(* Logix 5000 AddOnInstructionDefinition export Banner_DFG1_Param_v4; software revision 32.00; part 2 of 2 *)
(* tags used below, declared in another part *)
   DFG1 : Banner_DFG1_v2;
   Port_Data : Banner_IOL_Port_v4;
   Port : DINT;
   Local_Control : DINT;
   Command_Being_Processed : BOOL;
   Update_Archive : BOOL;
   Index_Write_Inprocess : DINT;
   Inprocess_Index : DINT;
(* Banner_DFG1_Param_v4, continued *)

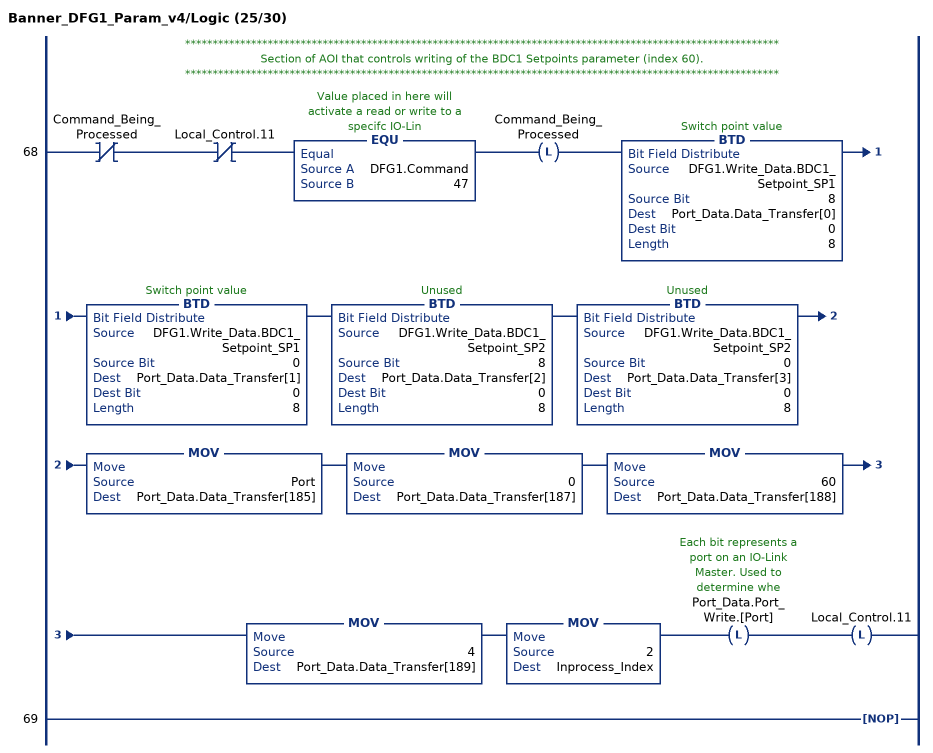
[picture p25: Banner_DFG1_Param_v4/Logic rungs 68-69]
   // ************************************************************************************************************
   // Section of AOI that controls writing of the BDC1 Setpoints parameter (index 60).
   // ************************************************************************************************************
   68: XIO(Command_Being_Processed)XIO(Local_Control.11)EQU(DFG1.Command,47)OTL(Command_Being_Processed)BTD(DFG1.Write_Data.BDC1_Setpoint_SP1,8,Port_Data.Data_Transfer[0],0,8)BTD(DFG1.Write_Data.BDC1_Setpoint_SP1,0,Port_Data.Data_Transfer[1],0,8)BTD(DFG1.Write_Data.BDC1_Setpoint_SP2,8,Port_Data.Data_Transfer[2],0,8)BTD(DFG1.Write_Data.BDC1_Setpoint_SP2,0,Port_Data.Data_Transfer[3],0,8)MOV(Port,Port_Data.Data_Transfer[185])MOV(0,Port_Data.Data_Transfer[187])MOV(60,Port_Data.Data_Transfer[188])MOV(4,Port_Data.Data_Transfer[189])MOV(2,Inprocess_Index)OTL(Port_Data.Port_Write.[Port])OTL(Local_Control.11);
   69: NOP();
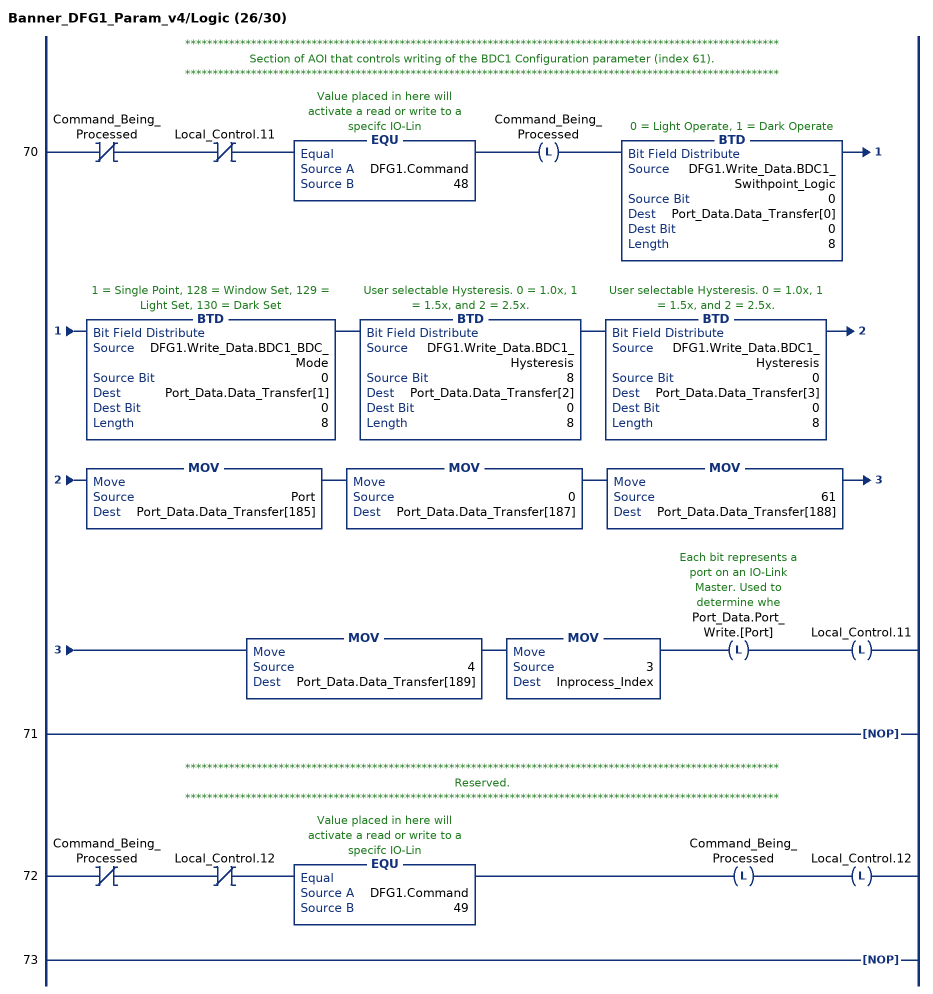
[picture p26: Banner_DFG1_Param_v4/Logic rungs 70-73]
   // ************************************************************************************************************
   // Section of AOI that controls writing of the BDC1 Configuration parameter (index 61).
   // ************************************************************************************************************
   70: XIO(Command_Being_Processed)XIO(Local_Control.11)EQU(DFG1.Command,48)OTL(Command_Being_Processed)BTD(DFG1.Write_Data.BDC1_Swithpoint_Logic,0,Port_Data.Data_Transfer[0],0,8)BTD(DFG1.Write_Data.BDC1_BDC_Mode,0,Port_Data.Data_Transfer[1],0,8)BTD(DFG1.Write_Data.BDC1_Hysteresis,8,Port_Data.Data_Transfer[2],0,8)BTD(DFG1.Write_Data.BDC1_Hysteresis,0,Port_Data.Data_Transfer[3],0,8)MOV(Port,Port_Data.Data_Transfer[185])MOV(0,Port_Data.Data_Transfer[187])MOV(61,Port_Data.Data_Transfer[188])MOV(4,Port_Data.Data_Transfer[189])MOV(3,Inprocess_Index)OTL(Port_Data.Port_Write.[Port])OTL(Local_Control.11);
   71: NOP();
   // ************************************************************************************************************
   // Reserved.
   // ************************************************************************************************************
   72: XIO(Command_Being_Processed)XIO(Local_Control.12)EQU(DFG1.Command,49)OTL(Command_Being_Processed)OTL(Local_Control.12);
   73: NOP();
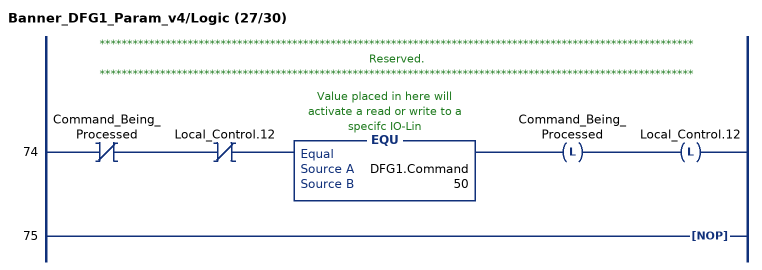
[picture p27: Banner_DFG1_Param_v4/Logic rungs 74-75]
   // ************************************************************************************************************
   // Reserved.
   // ************************************************************************************************************
   74: XIO(Command_Being_Processed)XIO(Local_Control.12)EQU(DFG1.Command,50)OTL(Command_Being_Processed)OTL(Local_Control.12);
   75: NOP();
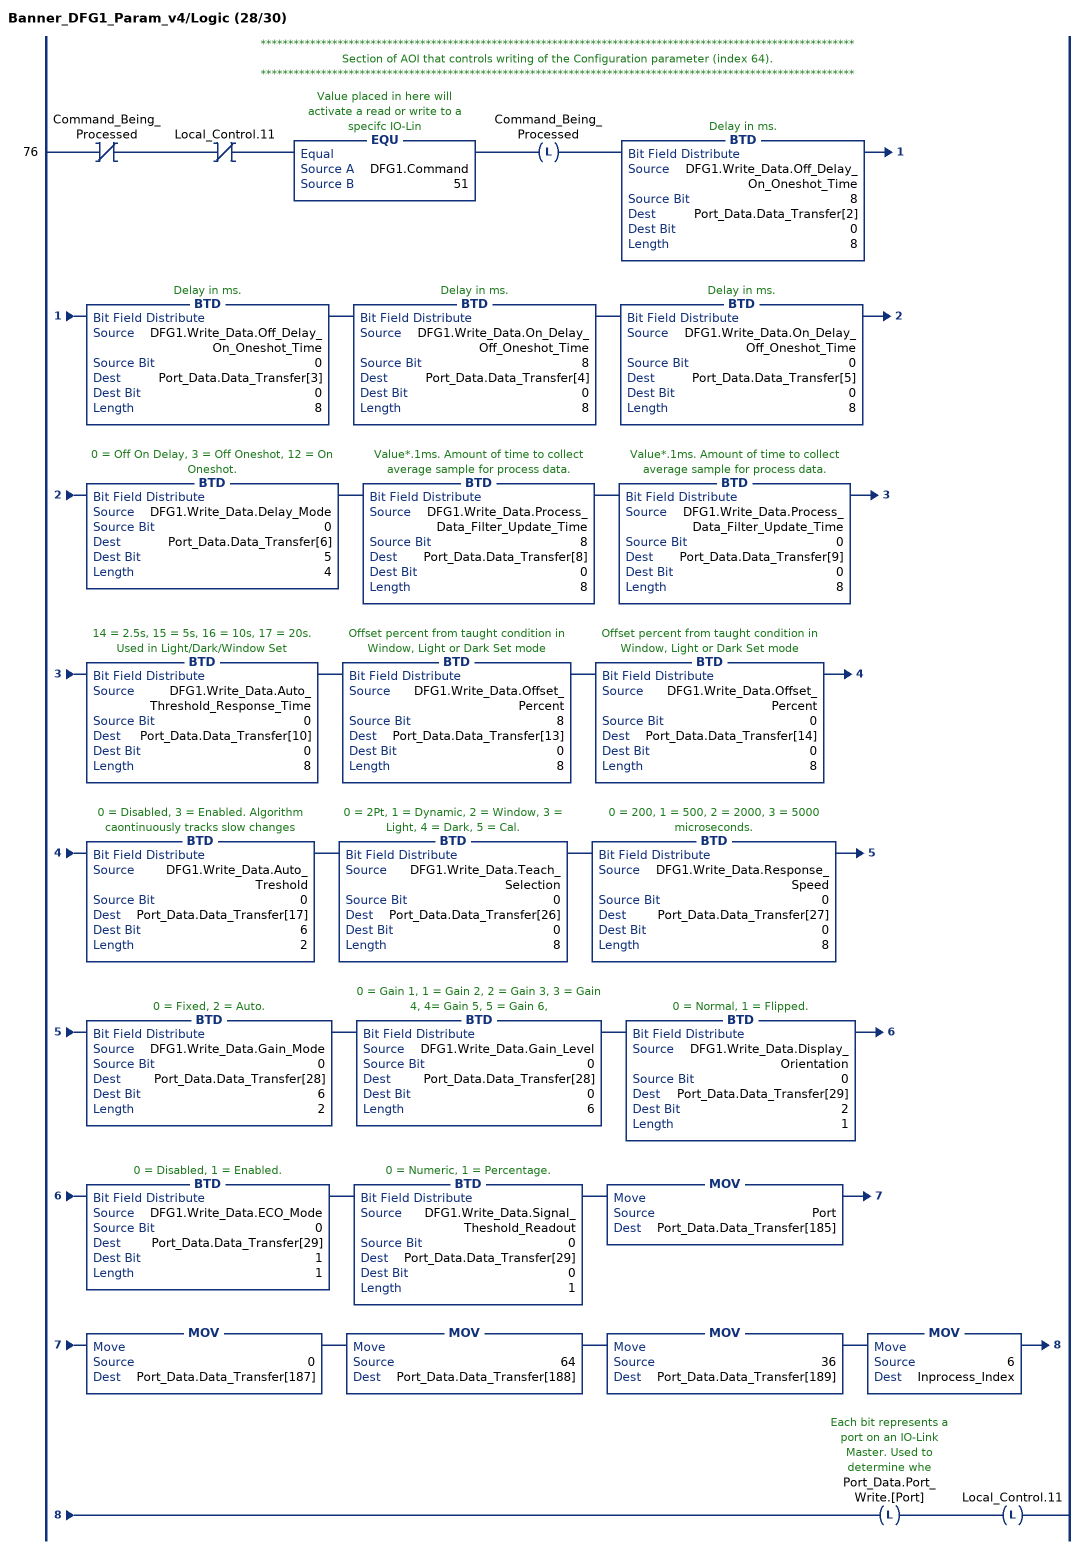
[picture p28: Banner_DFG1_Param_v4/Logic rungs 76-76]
   // ************************************************************************************************************
   // Section of AOI that controls writing of the Configuration parameter (index 64).
   // ************************************************************************************************************
   76: XIO(Command_Being_Processed)XIO(Local_Control.11)EQU(DFG1.Command,51)OTL(Command_Being_Processed)BTD(DFG1.Write_Data.Off_Delay_On_Oneshot_Time,8,Port_Data.Data_Transfer[2],0,8)BTD(DFG1.Write_Data.Off_Delay_On_Oneshot_Time,0,Port_Data.Data_Transfer[3],0,8)BTD(DFG1.Write_Data.On_Delay_Off_Oneshot_Time,8,Port_Data.Data_Transfer[4],0,8)BTD(DFG1.Write_Data.On_Delay_Off_Oneshot_Time,0,Port_Data.Data_Transfer[5],0,8)BTD(DFG1.Write_Data.Delay_Mode,0,Port_Data.Data_Transfer[6],5,4)BTD(DFG1.Write_Data.Process_Data_Filter_Update_Time,8,Port_Data.Data_Transfer[8],0,8)BTD(DFG1.Write_Data.Process_Data_Filter_Update_Time,0,Port_Data.Data_Transfer[9],0,8)BTD(DFG1.Write_Data.Auto_Threshold_Response_Time,0,Port_Data.Data_Transfer[10],0,8)BTD(DFG1.Write_Data.Offset_Percent,8,Port_Data.Data_Transfer[13],0,8)BTD(DFG1.Write_Data.Offset_Percent,0,Port_Data.Data_Transfer[14],0,8)BTD(DFG1.Write_Data.Auto_Treshold,0,Port_Data.Data_Transfer[17],6,2)BTD(DFG1.Write_Data.Teach_Selection,0,Port_Data.Data_Transfer[26],0,8)BTD(DFG1.Write_Data.Response_Speed,0,Port_Data.Data_Transfer[27],0,8)BTD(DFG1.Write_Data.Gain_Mode,0,Port_Data.Data_Transfer[28],6,2)BTD(DFG1.Write_Data.Gain_Level,0,Port_Data.Data_Transfer[28],0,6)BTD(DFG1.Write_Data.Display_Orientation,0,Port_Data.Data_Transfer[29],2,1)BTD(DFG1.Write_Data.ECO_Mode,0,Port_Data.Data_Transfer[29],1,1)BTD(DFG1.Write_Data.Signal_Theshold_Readout,0,Port_Data.Data_Transfer[29],0,1)MOV(Port,Port_Data.Data_Transfer[185])MOV(0,Port_Data.Data_Transfer[187])MOV(64,Port_Data.Data_Transfer[188])MOV(36,Port_Data.Data_Transfer[189])MOV(6,Inprocess_Index)OTL(Port_Data.Port_Write.[Port])OTL(Local_Control.11);
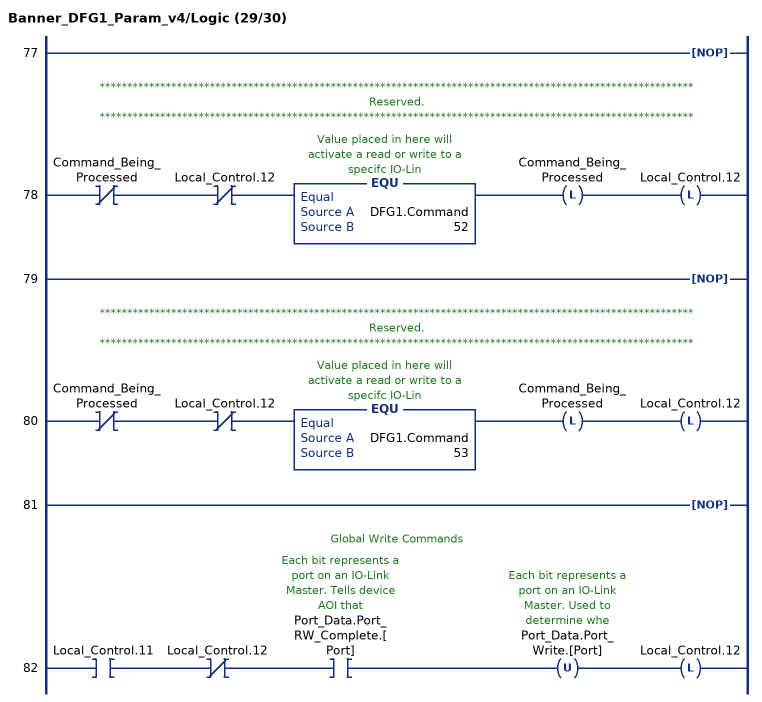
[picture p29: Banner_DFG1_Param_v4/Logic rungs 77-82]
   77: NOP();
   // ************************************************************************************************************
   // Reserved.
   // ************************************************************************************************************
   78: XIO(Command_Being_Processed)XIO(Local_Control.12)EQU(DFG1.Command,52)OTL(Command_Being_Processed)OTL(Local_Control.12);
   79: NOP();
   // ************************************************************************************************************
   // Reserved.
   // ************************************************************************************************************
   80: XIO(Command_Being_Processed)XIO(Local_Control.12)EQU(DFG1.Command,53)OTL(Command_Being_Processed)OTL(Local_Control.12);
   81: NOP();
   // Global Write Commands
   82: XIC(Local_Control.11)XIO(Local_Control.12)XIC(Port_Data.Port_RW_Complete.[Port])OTU(Port_Data.Port_Write.[Port])OTL(Local_Control.12);
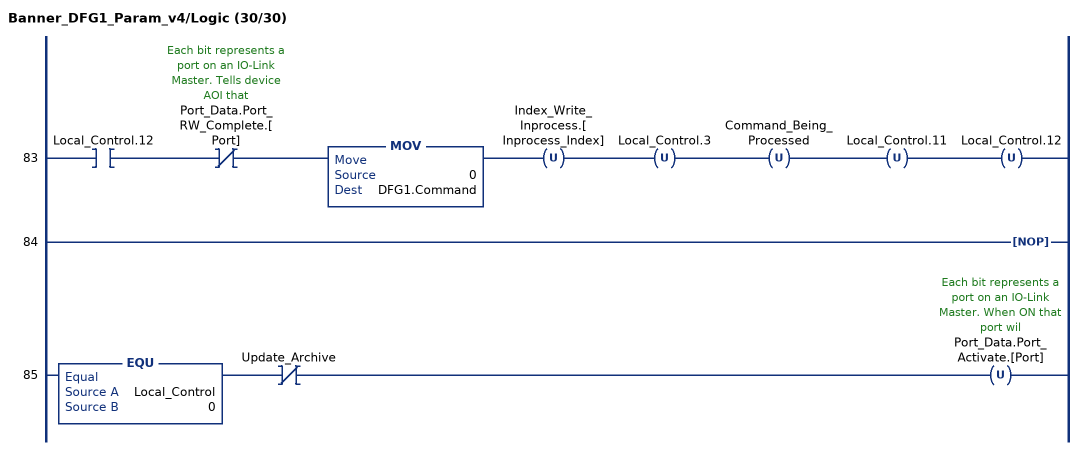
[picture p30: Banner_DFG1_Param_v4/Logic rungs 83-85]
   83: XIC(Local_Control.12)XIO(Port_Data.Port_RW_Complete.[Port])MOV(0,DFG1.Command)OTU(Index_Write_Inprocess.[Inprocess_Index])OTU(Local_Control.3)OTU(Command_Being_Processed)OTU(Local_Control.11)OTU(Local_Control.12);
   84: NOP();
   85: EQU(Local_Control,0)XIO(Update_Archive)OTU(Port_Data.Port_Activate.[Port]);
END_ROUTINE
END_ADD_ON_INSTRUCTION
